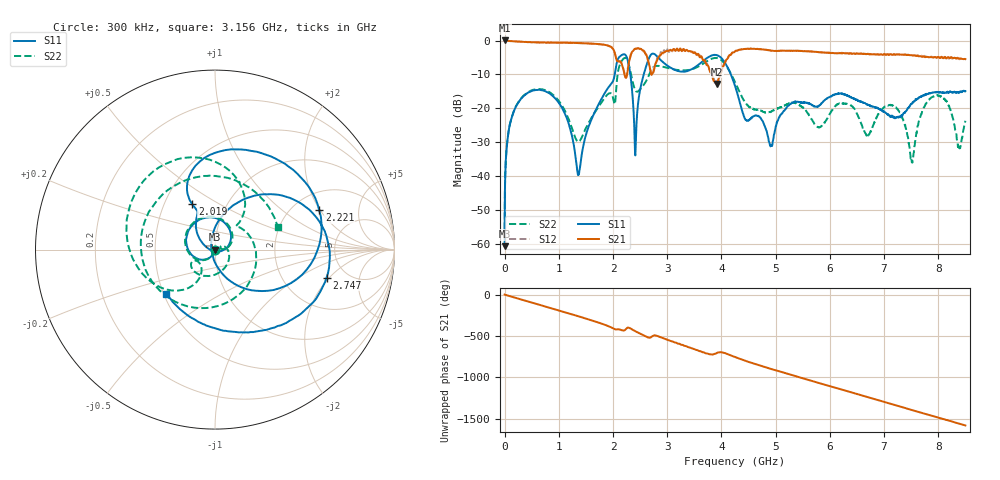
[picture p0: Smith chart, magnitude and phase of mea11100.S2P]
!Agilent Technologies,E5071B,MY42402595,A.08.01
!Date: Tue Jan 02 09:21:16 2001
!Data & Calibration Information:
!Freq	S11:SOLT2(ON)	S21:SOLT2(ON)	S12:SOLT2(ON)	S22:SOLT2(ON)
# Hz S dB R 50
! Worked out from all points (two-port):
!   1601 points, 300 kHz to 8.5 GHz, reference 50 ohm
!   highest |S21| = 0.03 dB at 300 kHz (marker M1); lowest = -12.8 dB at 3.91 GHz (marker M2)
!   |S21| within 3 dB of the highest: start of sweep to 2.018 GHz; 4.293 GHz to 4.913 GHz (619.8 MHz wide, 13.5 % of centre)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
!   lowest |S11| = -60.7 dB at 300 kHz (marker M3), VSWR 1.00, Z = 50.1 - j0.0101 ohm
!   |S11| at or under -10 dB: start of sweep to 2.032 GHz; 2.319 GHz to 2.567 GHz (248.5 MHz wide, 10.2 % of centre); 4.174 GHz to end of sweep
!   |S22| runs from -55.8 to -5.1 dB; largest |S21 - S12| = 0.066
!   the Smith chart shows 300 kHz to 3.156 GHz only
!   S11 on the Smith chart (normalised r, x): 300 kHz: 1.00, -0.00; 2.019 GHz: 0.69, +0.38; 2.221 GHz: 2.75, +1.96; 2.747 GHz: 3.52, -1.86; 3.156 GHz: 0.52, -0.29
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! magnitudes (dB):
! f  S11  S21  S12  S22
! 300 kHz  -60.7  0.0  0.0  -55.8
! 101.2 MHz  -24.5  -0.1  -0.2  -24.5
! 425.3 MHz  -15.4  -0.4  -0.5  -15.3
! 956.5 MHz  -17.4  -0.6  -0.6  -17.0
! 1.419 GHz  -34.0  -0.8  -0.8  -28.7
! 2.019 GHz  -11.0  -3.0  -3.1  -18.3
! 2.221 GHz  -4.1  -10.5  -10.2  -5.1
! 2.417 GHz  -31.4  -2.4  -2.4  -14.9
! 2.747 GHz  -3.9  -9.3  -8.8  -7.8
! 2.837 GHz  -5.1  -4.9  -4.9  -7.5
! 3.156 GHz  -8.7  -3.0  -3.0  -8.6
! 3.91 GHz  -4.3  -12.8  -12.1  -5.1
! 4.25 GHz  -13.4  -3.2  -3.2  -12.3
! 4.909 GHz  -31.1  -2.9  -2.9  -21.1
! 5.669 GHz  -19.1  -3.2  -3.2  -23.3
! 6.327 GHz  -16.3  -3.7  -3.7  -18.7
! 6.699 GHz  -18.9  -4.0  -3.9  -27.9
! 7.087 GHz  -22.0  -4.3  -4.1  -19.1
! 7.512 GHz  -18.7  -4.3  -4.3  -36.0
! 7.878 GHz  -15.4  -4.9  -4.8  -16.7
! 8.383 GHz  -15.4  -5.3  -5.5  -31.7
! 8.5 GHz  -14.9  -5.5  -5.5  -23.7
